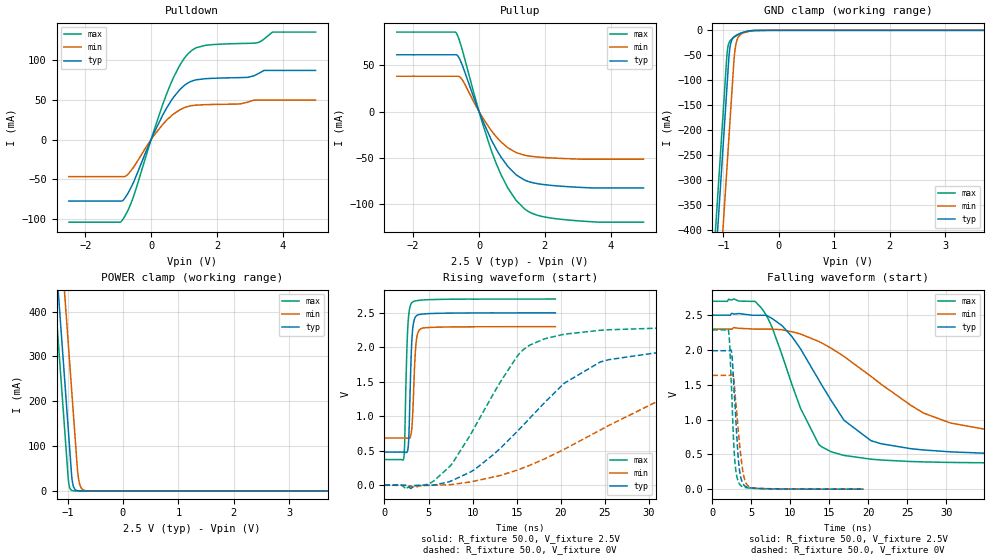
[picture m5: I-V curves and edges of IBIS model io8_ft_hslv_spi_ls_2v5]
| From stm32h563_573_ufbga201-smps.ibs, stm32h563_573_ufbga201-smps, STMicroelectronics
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[Model]   io8_ft_hslv_spi_ls_2v5
Model_type I/O
Polarity   Non-Inverting
Enable   Active-Low
| CAP_THRESHOLD on pad IOFT is "UDTCAPC" :
| Rising=20.0% of vddiom   Falling=80.0% of vddiom
| C_comp min and max val. don't necessarily correlate with the min and max pvt
| but are the smallest and greatest pad capacitance found.
| var   typ   min   max
C_comp   4.85178pF  4.77582pF  4.93402pF
|C_comp_pullup   3.10520pF  2.91250pF  2.94055pF
|C_comp_pulldown   1.74658pF  1.86332pF  1.99347pF
Vinl = 690.0mV
Vinh = 1.89V
Vmeas = 1.25V   | Reference voltage for timing measurements
Cref  = 50.0pF   | Timing specification test load capacitance value
Rref  = 100.0MOhm   | Timing specification test load resistance value
Vref  = 1.25V   | Timing specification test load voltage
[Model Spec]
| TIME_THRESHOLD on pin ZIV11 is "CMOS" :
| Rising=40.0% of vdd   Falling=60.0% of vdd
Vinl 989.80000mV 917.80000mV 1.06580V
Vinh 1.40320V 1.29620V 1.49120V
| variable   typ   min   max
[Temperature Range] 25.0 125.0 -40.0
| variable   typ   min   max
[Voltage Range] 2.5V 2.3V 2.7V
| variable   typ   min   max
[POWER Clamp Reference] 2.5V 2.3V 2.7V
| variable   typ   min   max
[GND Clamp Reference] 0V 0V 0V
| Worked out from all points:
|   slope of the pulldown table from 0 to 0.375 V, typ, clamps not added: 11.5 ohm
|   slope of the pullup table from 0 to 0.375 V, typ, clamps not added: 12.3 ohm
|   GND clamp passes 1 mA (typ) near -0.52 V on its own axis
|   POWER clamp passes 1 mA (typ) near -0.84 V on its own axis
|   rising waveform, R_fixture 50.0, V_fixture 2.5V: 20-80 % time 294ps typ, 331ps min, 293ps max; typ from 0.481 V to 2.5 V
|   falling waveform, R_fixture 50.0, V_fixture 2.5V: 20-80 % time 7.32ns typ, 13.2ns min, 4.82ns max; typ from 2.5 V to 0.481 V
|   rising waveform, R_fixture 50.0, V_fixture 0V: 20-80 % time 10ns typ, 16ns min, 6.46ns max; typ from 0 V to 1.99 V
|   falling waveform, R_fixture 50.0, V_fixture 0V: 20-80 % time 658ps typ, 862ps min, 531ps max; typ from 1.99 V to 0 V
[POWER Clamp]
-2.5V     2.708A     2.899A     2.597A
-1.23V    548.8mA    740.2mA    437.5mA
-1.16V    429.8mA    621.2mA    318.5mA
-1.07V    276.8mA    468.2mA    165.5mA
-1.03V    208.8mA    400.2mA    97.53mA
-980mV    123.8mA    315.2mA    17.95mA
-920mV    26.3mA     213.2mA    906uA
-880mV    5.543mA    145.2mA    123.7uA
-810mV    363.5uA    33.6mA     3.797uA
-770mV    76.62uA    10.47mA    518.9nA
-700mV    5.026uA    1.361mA    16.14nA
5V        0A         0A         0A
[GND Clamp]
-2.5V     -2.771A    -2.933A    -2.706A
-1.21V    -578.3mA   -739.7mA   -512.8mA
-950mV    -136.3mA   -297.7mA   -70.75mA
-930mV    -102.3mA   -263.7mA   -41.56mA
-900mV    -51.97mA   -212.7mA   -25.14mA
-880mV    -32.59mA   -178.7mA   -20.84mA
-850mV    -19.78mA   -127.7mA   -17.15mA
-810mV    -13.22mA   -60.17mA   -13.75mA
-780mV    -10.64mA   -30.96mA   -11.62mA
-730mV    -7.637mA   -13.21mA   -8.533mA
-430mV    -217.7uA   -562.2uA   -113.2uA
5V        7.27nA     1.305uA    342.4pA
| variable   typ   min   max
[Pullup Reference] 2.5V 2.3V 2.7V
| variable   typ   min   max
[Pulldown Reference] 0V 0V 0V
[Pullup]
-2.5V     61.27mA    38.13mA    85.8mA
-690mV    61.27mA    38.13mA    84.72mA
-610mV    58.21mA    37.94mA    78.19mA
-500mV    49.24mA    33.7mA     65.39mA
90mV      -7.973mA   -5.456mA   -10.93mA
510mV     -39.72mA   -26.68mA   -54.93mA
870mV     -59.1mA    -39.02mA   -82.25mA
1.13V     -68.42mA   -44.41mA   -96.07mA
1.38V     -73.93mA   -47.17mA   -105mA
1.77V     -77.87mA   -49.08mA   -112mA
2.42V     -80.46mA   -50.53mA   -116.1mA
5V        -82.5mA    -51.48mA   -119.5mA
[Pulldown]
-2.5V     -77.63mA   -46.84mA   -104.3mA
-870mV    -77.25mA   -46.84mA   -101.4mA
-550mV    -55.3mA    -35.88mA   -73.72mA
90mV      8.401mA    5.299mA    11.79mA
610mV     49.03mA    29.75mA    71.69mA
870mV     62.92mA    37.48mA    93.62mA
1.23V     73.63mA    42.72mA    112.2mA
1.64V     76.78mA    44.01mA    118.8mA
2.94V     78.48mA    47.15mA    121.4mA
3.24V     82.82mA    49.81mA    122.4mA
3.69V     87.21mA    49.81mA    135.6mA
5V        87.21mA    49.81mA    135.6mA
[Ramp]
dV/dt_r 1.19347V/9.48409ns 980.80819mV/15.69566ns 1.37307V/6.35644ns
dV/dt_f 1.21165V/6.829ns 969.25376mV/12.92409ns 1.39628V/4.54469ns
R_load = 50.0
| Removed startup time: 0s 0s 0s  .
| Removed end time: 19.4ns.
[Rising Waveform]
R_fixture   = 50.0
V_fixture   = 2.5V
V_fixture_min = 2.3V
V_fixture_max = 2.7V
0s        480.6mV    684.6mV    372.9mV
2.2ns     480.8mV    684.6mV    395mV
2.3ns     480.9mV    684.7mV    623.8mV
2.45ns    474.9mV    684.8mV    1.531V
2.65ns    513.9mV    680.4mV    2.293V
2.8ns     812.5mV    678.8mV    2.517V
3.15ns    2.182V     893.9mV    2.653V
3.55ns    2.446V     2.009V     2.674V
4.1ns     2.478V     2.266V     2.684V
19.4ns    2.499V     2.299V     2.699V
| Removed startup time: 0s 0s 0s  .
| Removed end time: 249.4ns.
[Falling Waveform]
R_fixture   = 50.0
V_fixture   = 2.5V
V_fixture_min = 2.3V
V_fixture_max = 2.7V
0s        2.5V       2.3V       2.7V
5.5ns     2.499V     2.3V       2.694V
8.9ns     2.354V     2.291V     1.941V
11.3ns    2.018V     2.229V     1.164V
13.65ns   1.569V     2.122V     642.9mV
16.9ns    988.8mV    1.905V     484.7mV
20.35ns   695.6mV    1.62V      430.9mV
30.55ns   536.3mV    949.9mV    384.2mV
50.9ns    488.8mV    739.4mV    373.7mV
249.4ns   480.6mV    684.6mV    372.9mV
| Removed startup time: 0s 0s 0s  .
| Removed end time: 249.4ns.
[Rising Waveform]
R_fixture   = 50.0
V_fixture   = 0V
V_fixture_min = 0V
V_fixture_max = 0V
0s        101.5nV    479.2nV    83.47nV
4.9ns     -679uV     -561.9uV   15.44mV
7.4ns     53.75mV    8.368mV    271.6mV
10.2ns    224.7mV    59.81mV    833.1mV
16.1ns    918.2mV    270.1mV    1.999V
20.4ns    1.479V     521mV      2.19V
24.5ns    1.788V     800.8mV    2.247V
35.6ns    1.954V     1.408V     2.283V
50.9ns    1.985V     1.591V     2.288V
249.4ns   1.989V     1.635V     2.288V
| Removed startup time: 0s 0s 0s  .
| Removed end time: 19.4ns.
[Falling Waveform]
R_fixture   = 50.0
V_fixture   = 0V
V_fixture_min = 0V
V_fixture_max = 0V
0s        1.989V     1.635V     2.288V
2.05ns    1.989V     1.635V     2.291V
2.2ns     1.99V      1.635V     2.119V
2.45ns    1.974V     1.643V     1.475V
2.85ns    1.309V     1.458V     450.5mV
3.3ns     479.1mV    870.1mV    116.5mV
3.6ns     192.1mV    528.9mV    57.33mV
4.2ns     44mV       117.5mV    24.37mV
5.15ns    15.05mV    18.15mV    13.77mV
19.4ns    335.4uV    564.3uV    235uV
